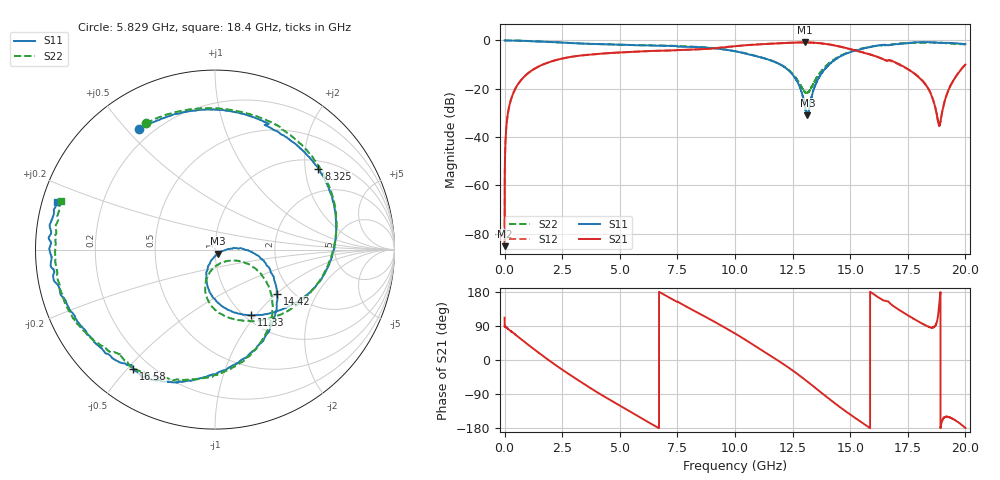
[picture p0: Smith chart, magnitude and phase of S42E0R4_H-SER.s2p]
! Created Wed Nov 25 21:22:49 2020
# khz S ma R 50
! 2 Port Network Data from SP1.SP block
! freq  magS11  angS11  magS21  angS21  magS12  angS12  magS22  angS22
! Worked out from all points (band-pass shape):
!   20001 points, 300 kHz to 20 GHz, reference 50 ohm
!   highest |S21| = -0.78 dB at 13.03 GHz (marker M1); lowest = -85.1 dB at 300 kHz (marker M2)
!   |S21| within 3 dB of the highest: 8.089695 GHz to 8.103106 GHz (13.41 MHz wide, 0.166 % of centre); 8.103 GHz to 15.1 GHz (6.995 GHz wide, 60.3 % of centre)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
!   lowest |S11| = -31.0 dB at 13.14 GHz (marker M3), VSWR 1.06, Z = 51.7 - j2.29 ohm
!   |S11| at or under -10 dB: 11.97 GHz to 14.08 GHz (2.105 GHz wide, 16.2 % of centre)
!   |S22| runs from -21.9 to 0.0 dB; largest |S21 - S12| = 0.015
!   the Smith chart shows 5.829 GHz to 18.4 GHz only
!   S11 on the Smith chart (normalised r, x): 5.829 GHz: 0.15, +0.54; 8.325 GHz: 1.22, +2.35; 11.33 GHz: 1.07, -0.95; 14.42 GHz: 1.67, -1.01; 16.58 GHz: 0.14, -0.52; 18.4 GHz: 0.04, +0.15
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300  0.9993 -0.3  5.546e-05 111.5  8.79e-05 70.6  1 -0.4
137300  0.9989 -6.8  0.0298 82.9  0.02998 82.8  0.9995 -6.7
520300  0.9932 -25.7  0.1118 64.4  0.1123 64.6  0.9933 -25.7
1815300  0.9402 -85.9  0.3392 4.0  0.3405 4.1  0.9366 -86.0
3334300  0.8643 -149.7  0.4889 -58.8  0.4891 -58.9  0.8636 -147.6
4525300  0.8281 166.0  0.5477 -103.6  0.5467 -103.6  0.832 167.4
5829300  0.7932 122.4  0.5907 -149.9  0.5898 -149.8  0.8027 118.7
6667300  0.7812 94.4  0.6127 -178.8  0.611 -179.1  0.7873 88.8
8325300  0.7308 38.0  0.6538 126.6  0.6491 126.5  0.7371 35.2
1.00003e7  0.598 -19.8  0.7605 69.9  0.7596 70.1  0.5995 -18.9
1.13303e7  0.419 -61.0  0.844 19.3  0.8453 19.6  0.4168 -70.4
1.24573e7  0.2068 -101.8  0.8968 -25.7  0.899 -26.1  0.2159 -104.8
1.30303e7  0.04506 -99.5  0.914 -51.6  0.9105 -51.8  0.08658 -79.9
1.31443e7  0.0282 -51.5  0.9085 -57.1  0.9083 -57.0  0.08293 -59.9
1.33343e7  0.0701 1.5  0.9012 -66.2  0.9007 -66.1  0.112 -32.9
1.44233e7  0.4248 -35.7  0.7696 -118.5  0.7746 -118.2  0.4401 -43.3
1.65773e7  0.8064 -124.3  0.3864 155.1  0.3777 155.7  0.794 -131.1
1.66673e7  0.7946 -126.2  0.3939 153.5  0.3841 153.9  0.7937 -133.1
1.84043e7  0.9192 162.9  0.09774 87.7  0.09876 88.1  0.9002 162.2
1.88763e7  0.8956 143.3  0.01755 153.9  0.0175 153.7  0.8995 143.6
1.93093e7  0.8868 125.6  0.1041 -151.2  0.1048 -151.6  0.8625 123.9
2e7  0.8449 95.3  0.3162 -179.4  0.321 -179.0  0.8264 86.7
